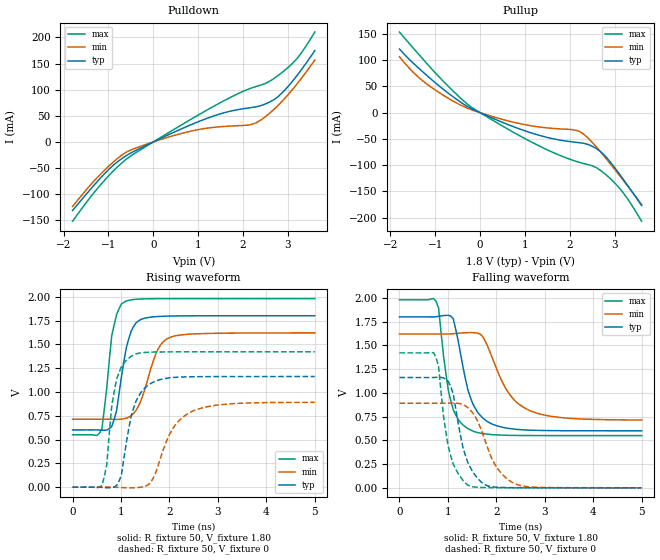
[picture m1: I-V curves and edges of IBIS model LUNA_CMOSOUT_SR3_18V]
[IBIS Ver]   3.2
[Comment Char]   |_char
[File name]   sg2016cbn_18v_b.ibs
[File Rev]   1.1
[Date]   2021/10/19 9:35:58
[Source]
[Notes]
[Disclaimer]
This information is for modeling purposes only, and is not guaranteed.
Property of SEIKO EPSON Corp.,
unauthorized reproduction and/or distribution is strictly prohibited.
[Copyright]
Copyright 2021, SEIKO EPSON Corp.
[Component]   2G005_2016
Si_location Pin
Timing_location Pin
[Manufacturer]   SEIKO EPSON Corp.
| 2016 PKG
[Package]
R_pkg   25m   NA   NA
L_pkg   0.25n   NA   NA
C_pkg   0.183p   NA   NA
[Pin] signal_name   model_name
1   OE   NC
2   GND   GND
3   OUT   LUNA_CMOSOUT_SR3_18V
4   VCC   POWER
| Models and submodels in the file (1): LUNA_CMOSOUT_SR3_18V (Output)
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[Model]   LUNA_CMOSOUT_SR3_18V
Model_type Output
Polarity Non-Inverting
Vmeas=0.90
C_comp   2.5p   2.0p   3.0p
[Temperature Range] 25   140   -40
[Voltage Range]   1.80   1.62   1.98
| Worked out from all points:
|   slope of the pulldown table from 0 to 0.27 V, typ, clamps not added: 24.5 ohm
|   slope of the pullup table from 0 to 0.27 V, typ, clamps not added: 26.4 ohm
|   falling waveform, R_fixture 50, V_fixture 1.80: 20-80 % time 354ps typ, 568ps min, 256ps max; typ from 1.8 V to 0.601 V
|   falling waveform, R_fixture 50, V_fixture 0: 20-80 % time 315ps typ, 459ps min, 256ps max; typ from 1.16 V to 0 V
|   rising waveform, R_fixture 50, V_fixture 1.80: 20-80 % time 242ps typ, 357ps min, 194ps max; typ from 0.601 V to 1.8 V
|   rising waveform, R_fixture 50, V_fixture 0: 20-80 % time 298ps typ, 493ps min, 197ps max; typ from 0 V to 1.16 V
[Pullup]
-1.8V     121.3mA    106.6mA    153.7mA
-1.5V     94.94mA    77.6mA     123.8mA
-1.2V     71.84mA    55.27mA    94.71mA
-700mV    36.45mA    26.85mA    49.42mA
-200mV    7.964mA    5.807mA    10.79mA
1.2V      -40.16mA   -25.82mA   -58.4mA
2.1V      -56.12mA   -32.76mA   -91.62mA
2.3V      -58.23mA   -40.3mA    -96.71mA
2.6V      -68.91mA   -66.22mA   -105.2mA
2.9V      -93.81mA   -97.22mA   -125.4mA
3.2V      -128.1mA   -129.9mA   -153.8mA
3.6V      -177.1mA   -174.9mA   -206.9mA
[Pulldown]
-1.8V     -131.2mA   -123.5mA   -151.7mA
-1.4V     -90.52mA   -82.16mA   -105.3mA
-1V       -53.18mA   -46.88mA   -65.06mA
-500mV    -21.07mA   -15.24mA   -26.54mA
500mV     20.11mA    13.3mA     26.01mA
1.2V      45.22mA    26.41mA    61.15mA
2.1V      64.74mA    32.11mA    100.3mA
2.4V      69.52mA    42.05mA    108.9mA
2.8V      87.99mA    71.35mA    128.2mA
3.1V      115.7mA    99.94mA    150mA
3.3V      137.9mA    121.5mA    170.2mA
3.6V      174.8mA    156.5mA    210.2mA
[Falling Waveform]
R_fixture=50
V_fixture=1.80
V_fixture_min=1.62
V_fixture_max=1.98
0s        1.8V       1.62V      1.98V
757.6ps   1.802V     1.62V      1.961V
808.1ps   1.805V     1.62V      1.894V
909.1ps   1.814V     1.619V     1.395V
1.061ns   1.809V     1.621V     917.2mV
1.414ns   1.03V      1.634V     623.8mV
1.818ns   697.2mV    1.495V     565.1mV
2.222ns   628.3mV    1.024V     553.6mV
2.677ns   607.6mV    816.6mV    551mV
5ns       600.6mV    714.4mV    550.3mV
[Falling Waveform]
R_fixture=50
V_fixture=0
V_fixture_min=0
V_fixture_max=0
0s        1.162V     891.2mV    1.421V
707.1ps   1.162V     891mV      1.421V
808.1ps   1.165V     891mV      1.279V
909.1ps   1.158V     891.1mV    758.6mV
1.01ns    1.118V     891.9mV    428.8mV
1.111ns   989.2mV    893.3mV    249.4mV
1.414ns   264.3mV    844.4mV    28.52mV
1.97ns    8.288mV    247.5mV    1.649mV
2.374ns   2.242mV    46.12mV    936uV
5ns       378.4uV    777.8uV    212.5uV
[Rising Waveform]
R_fixture=50
V_fixture=1.80
V_fixture_min=1.62
V_fixture_max=1.98
0s        600.5mV    713mV      550.3mV
606.1ps   597.6mV    713.3mV    612.6mV
808.1ps   636.6mV    712mV      1.588V
909.1ps   802.9mV    710.8mV    1.812V
1.111ns   1.468V     724.6mV    1.956V
1.212ns   1.64V      750.2mV    1.968V
1.364ns   1.746V     855.7mV    1.975V
1.717ns   1.79V      1.398V     1.979V
2.02ns    1.797V     1.574V     1.98V
5ns       1.8V       1.62V      1.98V
[Rising Waveform]
R_fixture=50
V_fixture=0
V_fixture_min=0
V_fixture_max=0
0s        0V         0V         0V
606.1ps   -2.769mV   198.6uV    16.35mV
707.1ps   -7.076mV   491.5uV    241.4mV
808.1ps   -5.879mV   -198.4uV   847.2mV
909.1ps   16.3mV     -2.216mV   1.134V
1.212ns   751.4mV    -7.551mV   1.375V
1.616ns   1.09V      49.81mV    1.418V
2.02ns    1.15V      571.5mV    1.42V
2.475ns   1.159V     797.1mV    1.421V
5ns       1.162V     890.7mV    1.421V
[Ramp]
R_load=50
dV/dt_r   6.969E-1/2.976E-10   5.344E-1/4.928E-10   8.526E-1/1.969E-10
dV/dt_f   7.196E-1/3.529E-10   5.434E-1/5.681E-10   8.578E-1/2.513E-10
|[End   LUNA_CMOSOUT_SR3_18V
